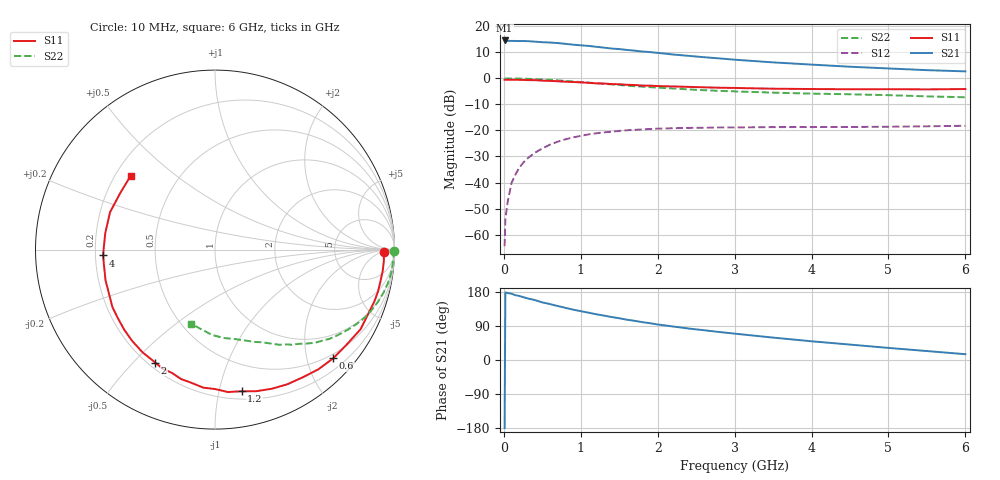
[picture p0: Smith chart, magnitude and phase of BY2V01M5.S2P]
! SIEMENS Small Signal Semiconductors
! BFY420
! Si NPN RF SIEGET Grounded Emitter Transistor in MICRO-X
! VCE = 2 V  IC = 1.5 mA
! Common Emitter S-Parameters:  October  1996
# GHz  S  MA  R  50
!  f  S11  S21  S12  S22
! GHz  MAG  ANG  MAG  ANG  MAG  ANG  MAG  ANG
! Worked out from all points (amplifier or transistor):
!   36 points, 10 MHz to 6 GHz, reference 50 ohm
!   highest |S21| = 14.6 dB at 10 MHz (marker M1)
!   |S21| within 3 dB of that: start of sweep to 1.371 GHz
!   unconditionally stable (mu >= 1): 4.252 GHz to end of sweep
!   at 250 MHz: K = 0.05, MSG = 23.4 dB, |S12| = -32.5 dB
!   at 1.4 GHz: K = 0.25, MSG = 16.0 dB, |S12| = -20.5 dB
!   at 6 GHz: K = 1.29, MAG = 7.2 dB, |S12| = -18.2 dB
!   S11 on the Smith chart (normalised r, x): 10 MHz: 32, -8; 600 MHz: 0.41, -2.51; 1.2 GHz: 0.26, -1.17; 2 GHz: 0.23, -0.58; 4 GHz: 0.23, -0.02; 6 GHz: 0.26, +0.35
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0.01  0.9427 -0.9  5.348 -179.5  0.0006 112.6  0.9979 -0.3
0.02  0.9412 -1.6  5.348 178.6  0.002 83.3  1 -0.7
0.05  0.9428 -3.8  5.238 176.7  0.0043 86.9  0.9962 -1.8
0.1  0.9419 -7.3  5.241 174.9  0.0098 87.7  0.9937 -3.7
0.15  0.9386 -10.8  5.226 171.0  0.0142 81.3  0.9924 -5.5
0.2  0.9377 -14.4  5.21 169.1  0.0192 81.3  0.9909 -7.2
0.3  0.9271 -21.6  5.192 163.0  0.0285 76.9  0.9818 -10.9
0.4  0.9243 -28.7  5.082 158.3  0.0371 72.9  0.9685 -14.5
0.5  0.9048 -35.7  4.95 152.0  0.0451 69.1  0.9532 -17.8
0.6  0.8949 -42.6  4.883 147.6  0.0534 65.1  0.9353 -21.2
0.8  0.8633 -55.5  4.603 137.6  0.0675 57.3  0.8939 -27.4
1.1  0.8217 -73.8  4.206 124.9  0.0841 47.6  0.8293 -35.4
1.2  0.8028 -79.4  4.04 120.8  0.0881 44.7  0.8082 -38.0
1.6  0.7532 -100.2  3.517 106.3  0.1008 34.6  0.7275 -46.1
2  0.712 -117.9  3.087 93.8  0.1084 27.0  0.6637 -52.7
2.2  0.7002 -125.3  2.874 88.4  0.1104 23.7  0.6405 -55.9
2.8  0.6618 -145.2  2.42 73.9  0.1141 16.7  0.5753 -63.7
3.5  0.6334 -164.4  2.029 59.1  0.116 11.4  0.5329 -71.8
4  0.6247 -177.0  1.839 49.4  0.1162 8.9  0.5095 -77.7
4.5  0.6183 171.5  1.674 40.7  0.1166 6.8  0.4955 -84.1
5.5  0.6149 149.1  1.439 23.6  0.1201 5.4  0.4516 -99.3
6  0.6245 138.8  1.363 15.3  0.123 5.3  0.4339 -108.0
